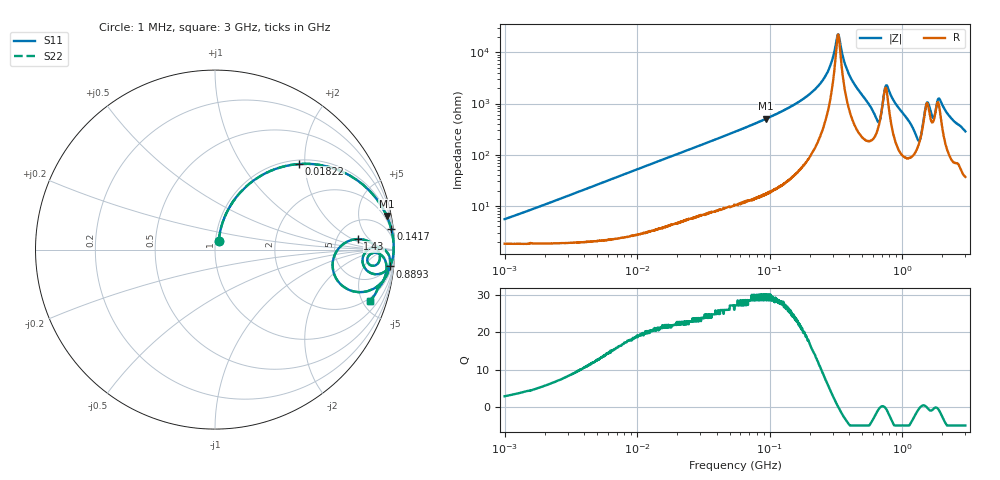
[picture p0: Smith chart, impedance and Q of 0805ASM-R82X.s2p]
!s-Parameter Generated by FASTRON Sdn. Bhd.
!FASTRON P/N : 0805ASM-R82X
!Keysight Technologies: E4991B_MY54100416_A.01.15
!Date: Fri Jun 19 14:53:43 2026
!Version  :Rev00  Fri Jun 19 14:53:43 2026
!Data & Calibration Information:
!Freq  S11  S21  S12  S22
!PortZ  Port1:50+j0  Port2:50+j0
!When reading reference impedance value at option line is always used.
! Remarks : This data is being provided solely for informational purposes.
# Hz S dB R 50
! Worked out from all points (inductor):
!   1601 points, 1 MHz to 3 GHz, reference 50 ohm
!   read as one part in series: L = 830 nH near 1.046 MHz
!   highest Q = 30.1 at 94.03 MHz (marker M1), where L = 855 nH
!   self-resonance near 328.5 MHz
!   S11 on the Smith chart (normalised r, x): 1 MHz: 1.04, +0.10; 18.22 MHz: 1.09, +1.87; 141.7 MHz: 2, +17; 889.3 MHz: 5, -20; 1.43 GHz: 8.05, +2.60; 3 GHz: 1.73, -5.66
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1000000  -25.30 67.8  -0.17 -2.9  -0.17 -2.9  -25.30 67.8
3804036  -14.40 73.4  -0.33 -11.0  -0.33 -11.0  -14.40 73.4
1.447069e7  -4.66 51.5  -2.12 -35.7  -2.12 -35.7  -4.66 51.5
1.821614e7  -3.50 45.5  -2.93 -41.9  -2.93 -41.9  -3.50 45.5
5.504702e7  -0.61 19.3  -9.62 -68.6  -9.62 -68.6  -0.61 19.3
9.402997e7  -0.22 11.1  -14.30 -76.9  -14.30 -76.9  -0.22 11.1
1.417323e8  -0.10 6.7  -18.70 -81.1  -18.70 -81.1  -0.10 6.7
2.083556e8  -0.05 3.4  -24.50 -82.9  -24.50 -82.9  -0.05 3.4
2.743666e8  -0.04 1.4  -32.40 -79.2  -32.40 -79.2  -0.04 1.4
3.285236e8  -0.04 0.0  -47.00 -2.3  -47.00 -2.3  -0.04 0.0
4.033367e8  -0.05 -1.6  -30.70 77.1  -30.70 77.1  -0.05 -1.6
6.455778e8  -1.11 -8.6  -14.70 45.5  -14.70 45.5  -1.11 -8.6
6.821091e8  -1.59 -1.6  -15.40 7.7  -15.40 7.7  -1.59 -1.6
7.50144e8  -0.37 -0.9  -27.10 19.2  -27.10 19.2  -0.37 -0.9
7.925923e8  -0.23 -2.7  -25.40 60.0  -25.40 60.0  -0.23 -2.7
8.892696e8  -0.19 -5.5  -20.20 74.2  -20.20 74.2  -0.19 -5.5
1.300759e9  -2.67 -15.8  -9.01 34.4  -9.01 34.4  -2.67 -15.8
1.430499e9  -1.96 4.2  -13.50 -16.1  -13.50 -16.1  -1.96 4.2
1.542004e9  -0.78 -1.0  -21.20 10.6  -21.20 10.6  -0.78 -1.0
1.712864e9  -1.34 -5.1  -15.70 27.3  -15.70 27.3  -1.34 -5.1
1.902655e9  -0.49 -3.1  -22.40 42.2  -22.40 42.2  -0.49 -3.1
3e9  -0.84 -18.4  -9.96 64.2  -9.96 64.2  -0.84 -18.4
